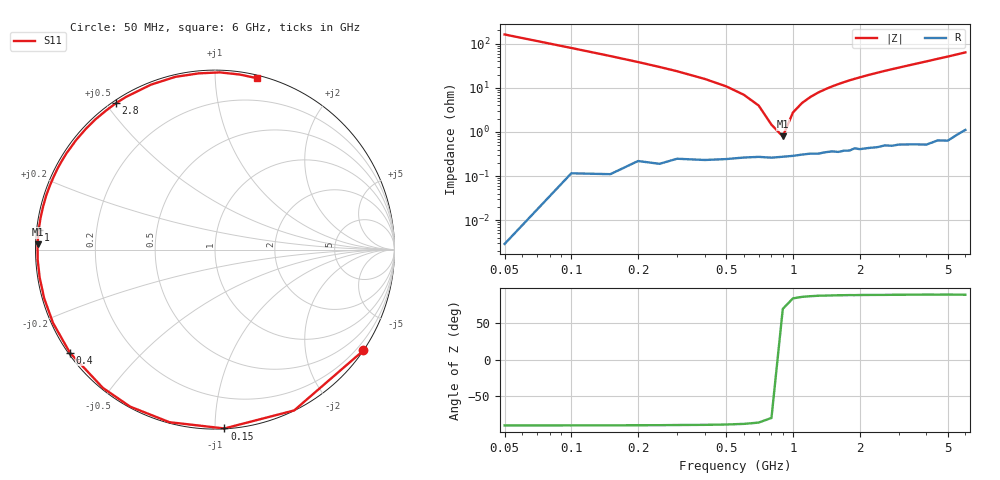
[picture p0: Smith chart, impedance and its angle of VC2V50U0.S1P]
! Infineon Technologies  Discrete & RF Semiconductors
! BBY 56-03
! Si Tuning Diode in SOD323
! VR = 2.5 V
! S-Parameters:  June  1999
# GHz  S  MA  R  50
!  f  S11
! GHz  MAG  ANG
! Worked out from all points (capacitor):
!   34 points, 50 MHz to 6 GHz, reference 50 ohm
!   read as one part to ground: C = 19.5 pF near 50 MHz
!   lowest |Z| = 791 mohm at 900 MHz (marker M1)
!   series resonance near 866 MHz, so ESL is about 1.7 nH
!   S11 on the Smith chart (normalised r, x): 50 MHz: 0.00, -3.25; 150 MHz: 0.00, -1.05; 400 MHz: 0.00, -0.32; 1 GHz: 0.01, +0.06; 2.8 GHz: 0.01, +0.53; 6 GHz: 0.02, +1.27
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0.05  1 -34.2
0.1  0.9987 -63.8
0.15  0.9979 -87.0
0.2  0.9945 -104.8
0.25  0.9944 -118.4
0.3  0.992 -129.0
0.4  0.9916 -144.6
0.5  0.9908 -155.6
0.6  0.9897 -164.1
0.7  0.9892 -170.9
0.8  0.9896 -176.7
0.9  0.9891 178.3
1  0.9886 173.7
1.1  0.9879 169.6
1.3  0.9875 162.2
1.6  0.9868 152.7
1.8  0.9862 147.0
2  0.9856 141.9
2.2  0.9851 137.0
2.4  0.985 132.5
2.8  0.9849 124.1
3  0.9846 120.2
3.5  0.9858 111.2
4  0.9874 102.9
4.5  0.986 95.3
5  0.9877 88.5
5.5  0.9852 82.0
6  0.9831 76.3
